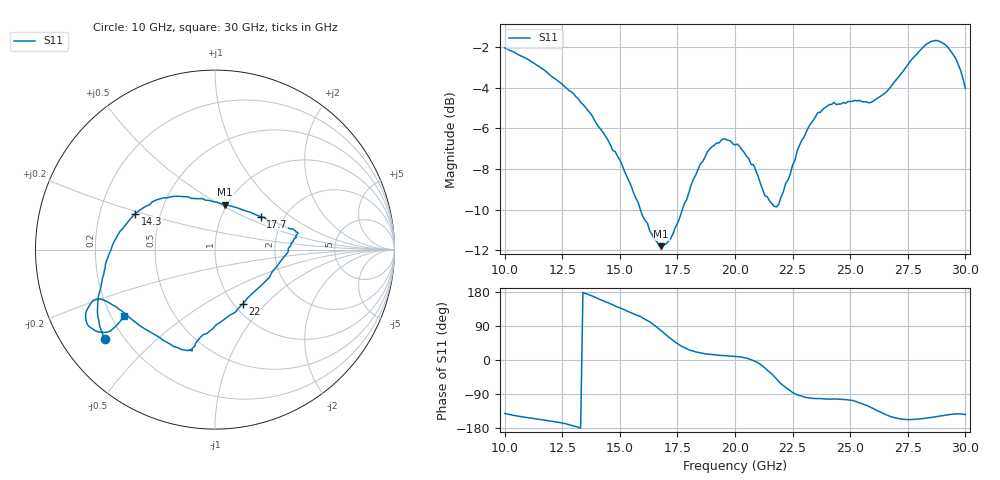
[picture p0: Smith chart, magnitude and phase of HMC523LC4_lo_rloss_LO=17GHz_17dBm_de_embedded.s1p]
!Hittite Microwave Corporation
!20 Alpha Rd
!Chelmsford, MA 01824
!Tel: 978-250-3343
!Fax: 978-250-3373
!Device: HMC523LC4, 10-30 GHz, GaAs MMIC Double-Balanced Mixer
!Misc: LO Return Loss with LO at 17 dBm, Room
# MHZ S MA R 50
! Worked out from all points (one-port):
!   201 points, 10 GHz to 30 GHz, reference 50 ohm
!   lowest |S11| = -11.8 dB at 16.8 GHz (marker M1), VSWR 1.69, Z = 49 + j26.3 ohm
!   |S11| at or under -10 dB: 15.89 GHz to 17.72 GHz (1.826 GHz wide, 10.9 % of centre)
!   S11 on the Smith chart (normalised r, x): 10 GHz: 0.13, -0.35; 14.3 GHz: 0.36, +0.19; 17.7 GHz: 1.53, +0.62; 22 GHz: 1.10, -0.75; 30 GHz: 0.25, -0.31
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10000  0.79 -141.1
11000  0.741 -152.1
12500  0.643 -166.3
13400  0.574 178.2
14300  0.487 155.8
15000  0.419 137.7
15800  0.329 116.8
16800  0.257 77.2
17500  0.292 43.5
17700  0.314 35.6
18800  0.438 15.3
19500  0.472 11.7
20000  0.456 9.3
20500  0.428 5.1
20900  0.395 -4.3
21700  0.322 -43.5
22000  0.34 -62.8
22500  0.407 -86.0
23300  0.516 -100.8
24300  0.58 -102.8
25000  0.583 -105.9
25700  0.582 -119.6
26800  0.638 -150.2
27500  0.718 -157.3
28200  0.797 -154.2
28700  0.824 -150.0
29500  0.756 -142.5
30000  0.628 -144.0
